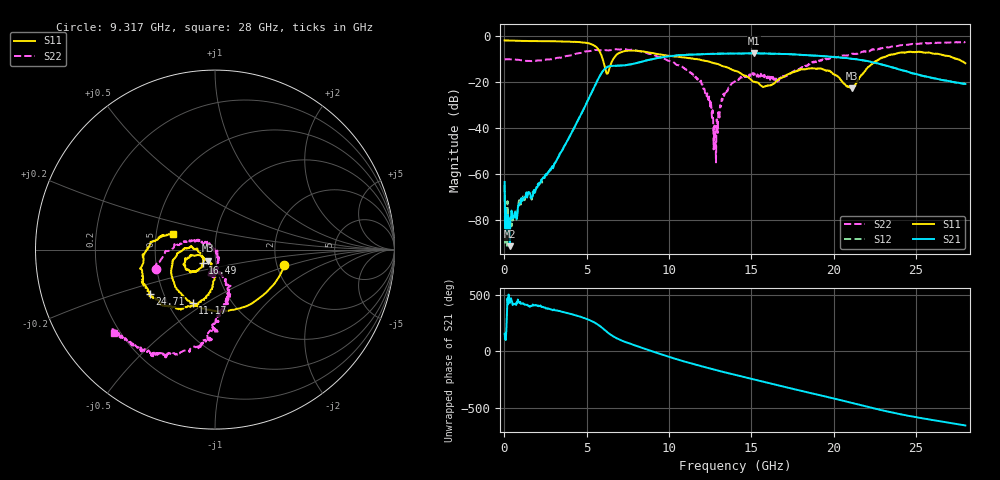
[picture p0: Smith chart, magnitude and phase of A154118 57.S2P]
!  2-Port S-parameters saved by WinCal
! VAR MeasName=S-Parameters (CALIBRATED_DATA) read from VNA (N5230A)
! VAR MeasDate=2015-9-10 14:39:31
! VAR NAME=A154118 57
! VAR FILENAME=A154118 57.S2P
! VAR DATE=2015-9-10 14:39:31
! VAR PHYS_PORTS=1,2
# Hz S DB R 50
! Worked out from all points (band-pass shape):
!   801 points, 10 MHz to 28 GHz, reference 50 ohm
!   highest |S21| = -7.69 dB at 15.16 GHz (marker M1); lowest = -91.3 dB at 324.9 MHz (marker M2)
!   |S21| within 3 dB of the highest: 8.686 GHz to 21.72 GHz (13.04 GHz wide, 85.7 % of centre)
!   lowest |S11| = -22.8 dB at 21.11 GHz (marker M3), VSWR 1.16, Z = 46.1 - j5.75 ohm
!   |S11| at or under -10 dB: 5.96 GHz to 6.626 GHz (666.3 MHz wide, 10.6 % of centre); 11.44 GHz to 22.81 GHz (11.38 GHz wide, 66.4 % of centre); 27.39 GHz to end of sweep
!   |S22| runs from -55.0 to -2.7 dB; largest |S21 - S12| = 0.008
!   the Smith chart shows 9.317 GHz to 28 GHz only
!   S11 on the Smith chart (normalised r, x): 9.317 GHz: 2.20, -0.44; 11.17 GHz: 0.66, -0.44; 16.49 GHz: 0.86, -0.13; 24.71 GHz: 0.42, -0.26; 28 GHz: 0.61, +0.12
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1e7  -2.15 179.7  -63.43 157.5  -64.72 -163.6  -10.43 179.8
3.248875e8  -2.20 175.2  -91.25 69.4  -85.48 112.0  -10.32 166.7
2.66905e9  -2.46 143.8  -59.31 17.0  -59.41 15.3  -10.36 75.9
4.698325e9  -3.01 98.3  -33.54 -57.7  -33.51 -58.0  -7.40 -14.8
5.677975e9  -5.75 36.8  -19.05 -122.9  -19.04 -123.0  -6.32 -54.6
6.1678e9  -15.65 -67.9  -14.01 179.9  -13.99 179.9  -6.34 -71.4
6.657625e9  -9.68 153.4  -13.12 128.8  -13.14 128.4  -6.02 -86.4
7.532312e9  -6.58 89.9  -12.64 72.6  -12.66 72.5  -6.20 -113.7
9.316675e9  -8.06 -12.4  -9.73 -16.1  -9.71 -16.0  -9.20 -161.4
9.351662e9  -8.09 -14.6  -9.71 -17.8  -9.68 -17.7  -9.19 -162.7
1.117101e10  -9.83 -112.6  -8.36 -100.2  -8.26 -100.7  -15.42 165.7
1.23256e10  -11.14 -152.0  -8.02 -146.0  -7.96 -146.7  -25.11 131.4
1.281542e10  -12.15 -163.5  -7.90 -164.6  -7.85 -165.3  -40.93 -25.5
1.323528e10  -13.21 -170.9  -7.85 179.7  -7.83 178.8  -28.06 -65.6
1.4005e10  -15.32 177.9  -7.83 151.4  -7.81 150.8  -19.90 -82.3
1.515959e10  -20.03 176.9  -7.69 110.6  -7.69 110.0  -16.47 -96.9
1.648911e10  -19.96 -132.9  -7.93 63.5  -7.88 62.9  -18.65 -94.1
1.869332e10  -14.14 -146.2  -8.67 -12.4  -8.68 -13.2  -11.46 -72.8
2.110746e10  -22.80 -120.9  -10.09 -96.7  -10.11 -97.7  -7.87 -87.8
2.334666e10  -8.55 -118.5  -13.36 -176.0  -13.35 -176.8  -5.15 -101.5
2.471118e10  -7.13 -145.9  -16.19 144.1  -16.29 143.1  -3.76 -114.4
2.8e10  -12.03 159.4  -20.96 63.2  -21.03 62.8  -2.73 -140.7
